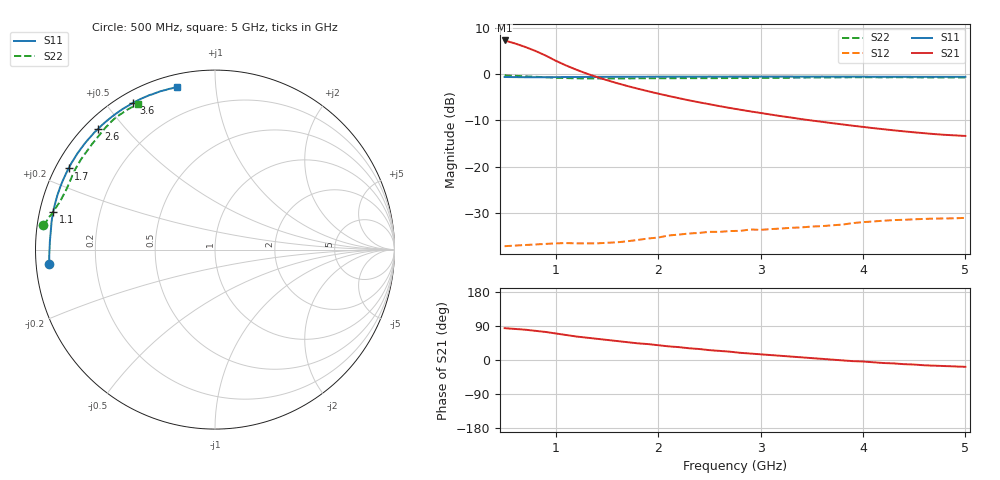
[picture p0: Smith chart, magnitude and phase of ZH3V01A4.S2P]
! SIEMENS Discrete & RF Semiconductors
! CLY38
! GaAs Power FET in MWP-35
! VDS = 3 V  ID = 1400 mA
! Common Source S-Parameters:  August  1998
# GHz  S  MA  R  50
!  f  S11  S21  S12  S22
! GHz  MAG  ANG  MAG  ANG  MAG  ANG  MAG  ANG
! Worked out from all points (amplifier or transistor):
!   46 points, 500 MHz to 5 GHz, reference 50 ohm
!   highest |S21| = 7.2 dB at 500 MHz (marker M1)
!   |S21| within 3 dB of that: start of sweep to 874.8 MHz
!   unconditionally stable (mu >= 1): 1.054 GHz to end of sweep
!   at 1.2 GHz: K = 1.18, MAG = 16.2 dB, |S12| = -36.6 dB
!   at 2.8 GHz: K = 1.80, MAG = 7.9 dB, |S12| = -33.9 dB
!   at 5 GHz: K = 2.19, MAG = 2.7 dB, |S12| = -31.1 dB
!   S11 on the Smith chart (normalised r, x): 500 MHz: 0.04, -0.04; 1.1 GHz: 0.04, +0.11; 1.7 GHz: 0.04, +0.26; 2.6 GHz: 0.04, +0.42; 3.6 GHz: 0.04, +0.59; 5 GHz: 0.06, +0.79
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0.5  0.927 -175.0  2.3 84.0  0.0138 16.0  0.966 172.0
0.7  0.922 180.0  1.96 80.0  0.0142 17.0  0.944 169.0
0.8  0.921 177.0  1.774 77.0  0.0144 16.0  0.932 168.0
1  0.924 170.0  1.387 70.0  0.0148 16.0  0.91 164.0
1.1  0.926 167.0  1.235 66.0  0.0149 16.0  0.902 162.0
1.2  0.927 164.0  1.112 62.0  0.0148 16.0  0.897 160.0
1.3  0.929 161.0  1.01 59.0  0.0148 16.0  0.894 159.0
1.5  0.931 156.0  0.856 53.0  0.015 16.0  0.893 156.0
1.7  0.933 151.0  0.74 47.0  0.0156 15.0  0.895 153.0
2  0.935 145.0  0.613 39.0  0.0171 15.0  0.899 148.0
2.3  0.936 139.0  0.519 31.0  0.0189 14.0  0.9 144.0
2.6  0.936 134.0  0.449 24.0  0.0197 14.0  0.901 141.0
2.8  0.937 131.0  0.411 19.0  0.0202 12.0  0.903 139.0
2.9  0.937 129.0  0.394 17.0  0.0209 12.0  0.904 137.0
3  0.937 127.0  0.379 15.0  0.0207 11.0  0.906 136.0
3.5  0.936 120.0  0.314 5.0  0.0225 8.0  0.914 131.0
3.6  0.937 119.0  0.304 3.0  0.0227 7.0  0.916 130.0
3.9  0.935 114.0  0.276 -3.0  0.0245 6.0  0.92 127.0
4.3  0.933 109.0  0.246 -9.0  0.0264 3.0  0.92 123.0
4.7  0.93 105.0  0.224 -15.0  0.0274 0.0  0.918 119.0
4.9  0.931 103.0  0.217 -17.0  0.0276 -1.0  0.918 118.0
5  0.931 103.0  0.214 -18.0  0.0279 -1.0  0.918 118.0
